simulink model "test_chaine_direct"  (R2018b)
settings: Solver=VariableStepAuto  StartTime=0.0  StopTime=10.0  RelTol=1e-3
undefined symbols (not defined in the file): AB2, AB_INV, ENV, MCC, RED, VEH

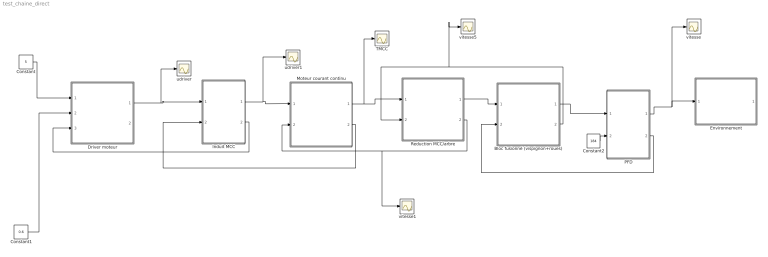
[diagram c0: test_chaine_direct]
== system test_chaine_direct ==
  Bloc fusionné (vispignon+roues) : Subsystem  AncestorBlock=simulink/REM/EC Elec  mask(Hacheur){}
  Constant : Constant  Value=5
  Constant1 : Constant  Value=0.6
  Constant2 : Constant  Value=184
  Driver moteur : Subsystem  AncestorBlock=simulink/REM/EC Elec  mask(Hacheur){}
  Environnement : Subsystem  AncestorBlock=simulink/REM/SE
  Induit MCC : Subsystem  AncestorBlock=simulink/REM/EA  mask(CM){}
  Moteur courant continu : Subsystem  AncestorBlock=simulink/REM/EC EM
  PFD : Subsystem  AncestorBlock=simulink/REM/EA  mask(CM){}
  Reduction MCC/arbre : Subsystem  AncestorBlock=simulink/REM/EC Elec  mask(Hacheur){}
  TMCC : Scope
  udriver : Scope
  udriver1 : Scope
  vitesse : Scope
  vitesse1 : Scope
  vitesse5 : Scope
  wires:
  PFD/2(vvehicule) -> Bloc fusionné (vispignon+roues)/2(v_vehicule)
  Bloc fusionné (vispignon+roues)/2(Omega_arbre) -> vitesse5/1, Reduction MCC/arbre/2(Omega)
  Constant/1 -> Driver moteur/1(Usel)
  Bloc fusionné (vispignon+roues)/1(Tred2) -> PFD/1(Tred2)
  Environnement/1(F_res) -> ?
  Constant1/1 -> Driver moteur/2(reg_uP)
  Reduction MCC/arbre/1(Tred) -> Bloc fusionné (vispignon+roues)/1(Tred)
  Reduction MCC/arbre/2(OmegaMCC) -> vitesse1/1, Moteur courant continu/2(OmegaMCC)
  Driver moteur/1(Udriver) -> udriver/1, Induit MCC/1(Udriver)
  PFD/1(v_vehicule) -> Environnement/1(V_vehicule), vitesse/1
  Moteur courant continu/1(TMCC) -> TMCC/1, Reduction MCC/arbre/1(TMCC)
  Moteur courant continu/2(UMCC) -> Induit MCC/2(UMCC)
  Induit MCC/1(I_ind) -> udriver1/1, Moteur courant continu/1(I_ind)
  Induit MCC/2(Iind) -> Driver moteur/3(Iind)
  Constant2/1 -> PFD/2(Fres)

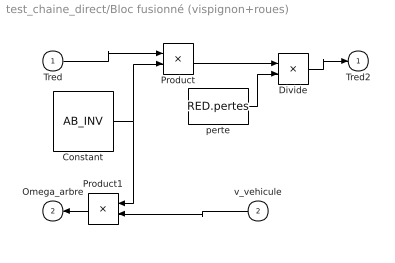
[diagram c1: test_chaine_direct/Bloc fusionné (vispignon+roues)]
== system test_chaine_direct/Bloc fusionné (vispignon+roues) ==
  Tred : Inport
  v_vehicule : Inport  Port=2
  Constant : Constant  Value=AB_INV
  Divide : Product  Inputs=*/
  Product : Product
  Product1 : Product
  perte : Constant  Value=RED.pertes
  Tred2 : Outport  InitialOutput=0
  Omega_arbre : Outport  Port=2  InitialOutput=0
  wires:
  Tred/1 -> Product/1
  Product/1 -> Divide/1
  Product1/1 -> Omega_arbre/1
  v_vehicule/1 -> Product1/2
  Constant/1 -> Product1/1, Product/2
  perte/1 -> Divide/2
  Divide/1 -> Tred2/1

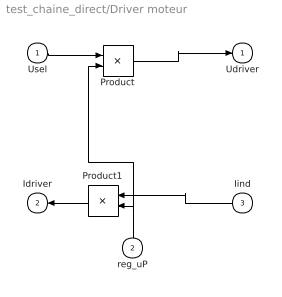
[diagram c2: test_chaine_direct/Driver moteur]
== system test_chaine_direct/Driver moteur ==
  Usel : Inport
  reg_uP : Inport  Port=2
  Iind : Inport  Port=3
  Product : Product
  Product1 : Product
  Udriver : Outport  InitialOutput=0
  Idriver : Outport  Port=2  InitialOutput=0
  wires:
  reg_uP/1 -> Product1/2, Product/2
  Usel/1 -> Product/1
  Product/1 -> Udriver/1
  Iind/1 -> Product1/1
  Product1/1 -> Idriver/1

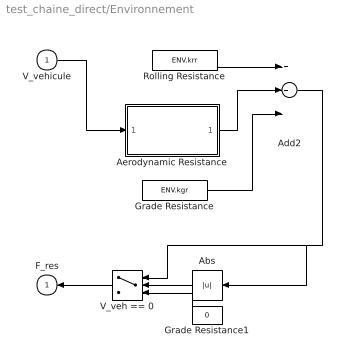
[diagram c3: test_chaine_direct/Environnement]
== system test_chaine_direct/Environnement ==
  V_vehicule : Inport
  Abs : Abs
  Add2 : Sum  Inputs=3
  Aerodynamic Resistance : Subsystem
  Grade Resistance : Constant  Value=ENV.kgr
  Grade Resistance1 : Constant  Value=0
  Rolling Resistance : Constant  Value=ENV.krr
  V_veh == 0 : Switch  Threshold=0.1
  F_res : Outport  InitialOutput=0
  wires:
  Grade Resistance1/1 -> V_veh == 0/3
  Abs/1 -> V_veh == 0/2
  Rolling Resistance/1 -> Add2/1
  Aerodynamic Resistance/1(F_ar) -> Add2/2
  V_veh == 0/1 -> F_res/1
  Grade Resistance/1 -> Add2/3
  Add2/1 -> Abs/1, V_veh == 0/1
  V_vehicule/1 -> Aerodynamic Resistance/1(V_veh)

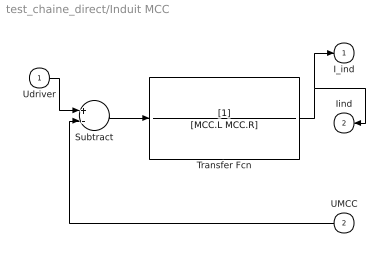
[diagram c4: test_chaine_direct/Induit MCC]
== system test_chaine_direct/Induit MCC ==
  Udriver : Inport
  UMCC : Inport  Port=2
  Subtract : Sum  Inputs=+-
  Transfer Fcn : TransferFcn  Denominator=[MCC.L MCC.R]
  I_ind : Outport  InitialOutput=0
  Iind : Outport  Port=2  InitialOutput=0
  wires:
  Udriver/1 -> Subtract/1
  UMCC/1 -> Subtract/2
  Transfer Fcn/1 -> Iind/1, I_ind/1
  Subtract/1 -> Transfer Fcn/1

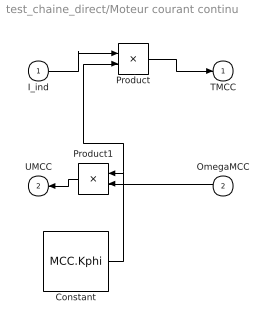
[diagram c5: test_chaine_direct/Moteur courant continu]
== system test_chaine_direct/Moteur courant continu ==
  I_ind : Inport
  OmegaMCC : Inport  Port=2
  Constant : Constant  Value=MCC.Kphi
  Product : Product
  Product1 : Product
  TMCC : Outport  InitialOutput=0
  UMCC : Outport  Port=2  InitialOutput=0
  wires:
  I_ind/1 -> Product/1
  Constant/1 -> Product1/1, Product/2
  Product/1 -> TMCC/1
  OmegaMCC/1 -> Product1/2
  Product1/1 -> UMCC/1

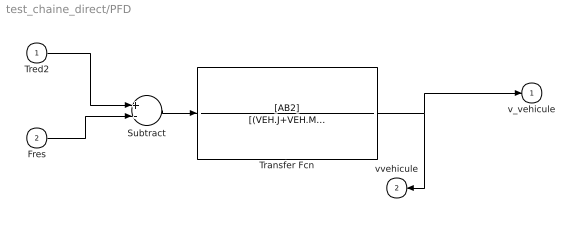
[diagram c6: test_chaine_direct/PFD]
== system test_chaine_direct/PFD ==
  Tred2 : Inport
  Fres : Inport  Port=2
  Subtract : Sum  Inputs=+-
  Transfer Fcn : TransferFcn  Numerator=[AB2]  Denominator=[(VEH.J+VEH.MPLUS*AB2) VEH.f]
  v_vehicule : Outport  InitialOutput=0
  vvehicule : Outport  Port=2  InitialOutput=0
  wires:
  Fres/1 -> Subtract/2
  Tred2/1 -> Subtract/1
  Transfer Fcn/1 -> v_vehicule/1, vvehicule/1
  Subtract/1 -> Transfer Fcn/1

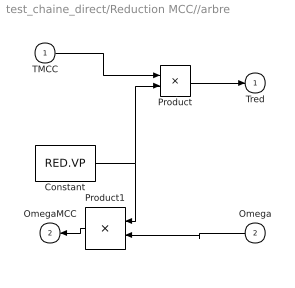
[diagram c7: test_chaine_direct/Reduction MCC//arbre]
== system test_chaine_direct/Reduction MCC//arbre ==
  TMCC : Inport
  Omega : Inport  Port=2
  Constant : Constant  Value=RED.VP
  Product : Product
  Product1 : Product
  Tred : Outport  InitialOutput=0
  OmegaMCC : Outport  Port=2  InitialOutput=0
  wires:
  TMCC/1 -> Product/1
  Product/1 -> Tred/1
  Product1/1 -> OmegaMCC/1
  Omega/1 -> Product1/2
  Constant/1 -> Product/2, Product1/1

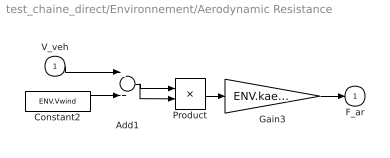
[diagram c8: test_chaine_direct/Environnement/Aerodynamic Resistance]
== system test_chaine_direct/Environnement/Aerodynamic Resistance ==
  V_veh : Inport
  Add1 : Sum
  Constant2 : Constant  Value=ENV.Vwind
  Gain3 : Gain  Gain=ENV.kaero
  Product : Product
  F_ar : Outport  InitialOutput=0
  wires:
  Gain3/1 -> F_ar/1
  Product/1 -> Gain3/1
  Add1/1 -> Product/1, Product/2
  Constant2/1 -> Add1/2
  V_veh/1 -> Add1/1
